(* 	
	Program Name: 	ACS_INITIALIZATION_NOBRAKE
	Purpose:		Example of Initialization of Drive
	When Executed:	Enables drive and performs homing routine if there are no faults
*)
PROGRAM ACS_INITIALIZATION_NOBRAKE
VAR_IN_OUT
	Axis:ACS_DRIVE_TYPE;
END_VAR

//If there are faults or if the drive is enabled and homed, this should just fall through

//Only if there are no faults...
IF Axis.InputFaultActive < 1 THEN

	//If we are not enabled, then enable
	IF Axis.InputStatusDriveEnabled < 1 THEN
		ACS_CMD_ENABLE(Axis:=Axis);

	//If we are enabled, but not homed, then home
	ELSE 
		IF Axis.InputStatusDriveHomed < 1 THEN
			ACS_CMD_HOME(Axis:=Axis);
		END_IF
	END_IF
	
END_IF

END_PROGRAM
